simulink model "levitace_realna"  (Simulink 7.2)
settings: Solver=ode5  SolverMode=SingleTasking  StartTime=0.0  StopTime=inf  MaxStep=0.001  RelTol=1e-3  AbsTol=1e-5
PreLoadFcn:
  | Ts=2e-3;
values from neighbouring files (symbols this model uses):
  Kreg3 = lqg(sys,0.0001*eye(4),QMV,10000)    [podklad.m]
undefined symbols (not defined in the file or in its folder): Humusoft, MF624, to, V
libraries: rtlib x3, simulink x2

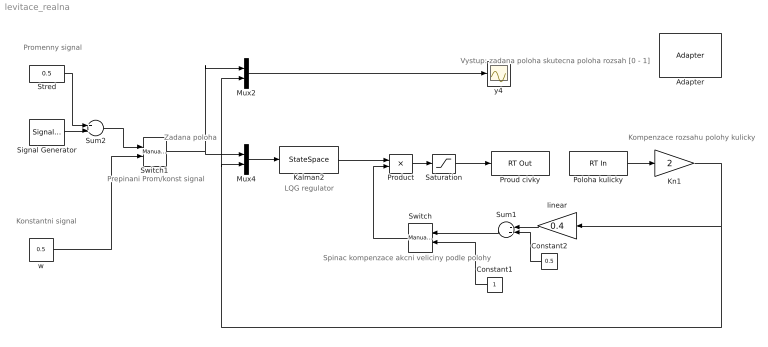
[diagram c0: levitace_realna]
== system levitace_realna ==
  note: Promenny signal
  note: Konstantni signal
  note: Prepinani Prom/konst signal
  note: Spinac kompenzace akcni veliciny podle polohy
  note: LQG regulator
  note: Kompenzace rozsahu polohy kulicky
  note: Zadana poloha
  note: Vystup: zadana poloha skutecna poloha rozsah [0 - 1]
  Adapter : rtlib/Adapter  SystemSampleTime=-1  DriverName=Humusoft/MF624  DriverAddress=4294967295  DriverOptions=0
  Constant1 : Constant  Orientation=left  OutDataType=sfix(16)  OutScaling=2^0
  Constant2 : Constant  Orientation=left  Value=0.5  OutDataType=sfix(16)  OutScaling=2^0
  Kalman2 : StateSpace  A=Kreg3.a  B=Kreg3.b  C=Kreg3.c  D=Kreg3.d
  Kn1 : Gain  Gain=2  ParameterDataType=sfix(16)  ParameterScaling=2^0  OutDataType=sfix(16)  OutScaling=2^0
  Mux2 : Mux  Inputs=2
  Mux4 : Mux  Inputs=2
  Poloha kulicky : rtlib/RT In  SampleTime=Ts  Adapter=Adapter  IOClass=Analog Input  Channels=1  SLDataType=double  MaxMissedTicks=2000  ShowMissedTicks=off  YieldWhenWaiting=on  AIORange=-10 to 10 V  AIOUnits=Normalized bipolar  DIOMode=Bit  CIReset=never  CIEdge=rising  CIGate=none  EIQuadrature=quadruple  EIIndexPulse=reset  EIFilterFrequency=Inf  OIOParameters=[]
  Product : Product  OutDataType=sfix(16)  OutScaling=2^0
  Proud civky : rtlib/RT Out  SampleTime=Ts  Adapter=Adapter  IOClass=Analog Output  Channels=1  InitialValue=[]  FinalValue=[]  MaxMissedTicks=1000  ShowMissedTicks=off  YieldWhenWaiting=on  AIORange=-10 to 10 V  AIOUnits=Normalized bipolar  DIOMode=Bit  OIOParameters=[]
  Saturation : Saturate  UpperLimit=1  LowerLimit=0
  Signal Generator : SignalGenerator  WaveForm=square  Amplitude=0.200  Frequency=0.5
  Stred : Constant  Value=0.5  OutDataType=sfix(16)  OutScaling=2^0
  Sum1 : Sum  Orientation=left  Inputs=-+  OutDataType=sfix(16)  OutScaling=2^0
  Sum2 : Sum  OutDataType=sfix(16)  OutScaling=2^0
  Switch : simulink/Signal Routing/Manual Switch  Orientation=left  SystemSampleTime=-1  sw=1  action=0  varsize=off
  Switch1 : simulink/Signal Routing/Manual Switch  SystemSampleTime=-1  sw=1  action=0  varsize=off
  linear : Gain  Orientation=left  Gain=0.4  ParameterDataType=sfix(16)  ParameterScaling=2^0  OutDataType=sfix(16)  OutScaling=2^0
  w : Constant  Value=0.5  OutDataType=sfix(16)  OutScaling=2^0
  y4 : Scope
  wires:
  Kalman2/1 -> Product/1
  Product/1 -> Saturation/1
  linear/1 -> Sum1/1
  Constant2/1 -> Sum1/2
  Saturation/1 -> Proud civky/1
  Sum1/1 -> Switch/1
  Switch/1 -> Product/2
  Stred/1 -> Sum2/1
  Signal Generator/1 -> Sum2/2
  w/1 -> Switch1/2
  Poloha kulicky/1 -> Kn1/1
  Kn1/1 -> linear/1, Mux4/2, Mux2/2
  Sum2/1 -> Switch1/1
  Switch1/1 -> Mux4/1, Mux2/1
  Mux4/1 -> Kalman2/1
  Constant1/1 -> Switch/2
  Mux2/1 -> y4/1
